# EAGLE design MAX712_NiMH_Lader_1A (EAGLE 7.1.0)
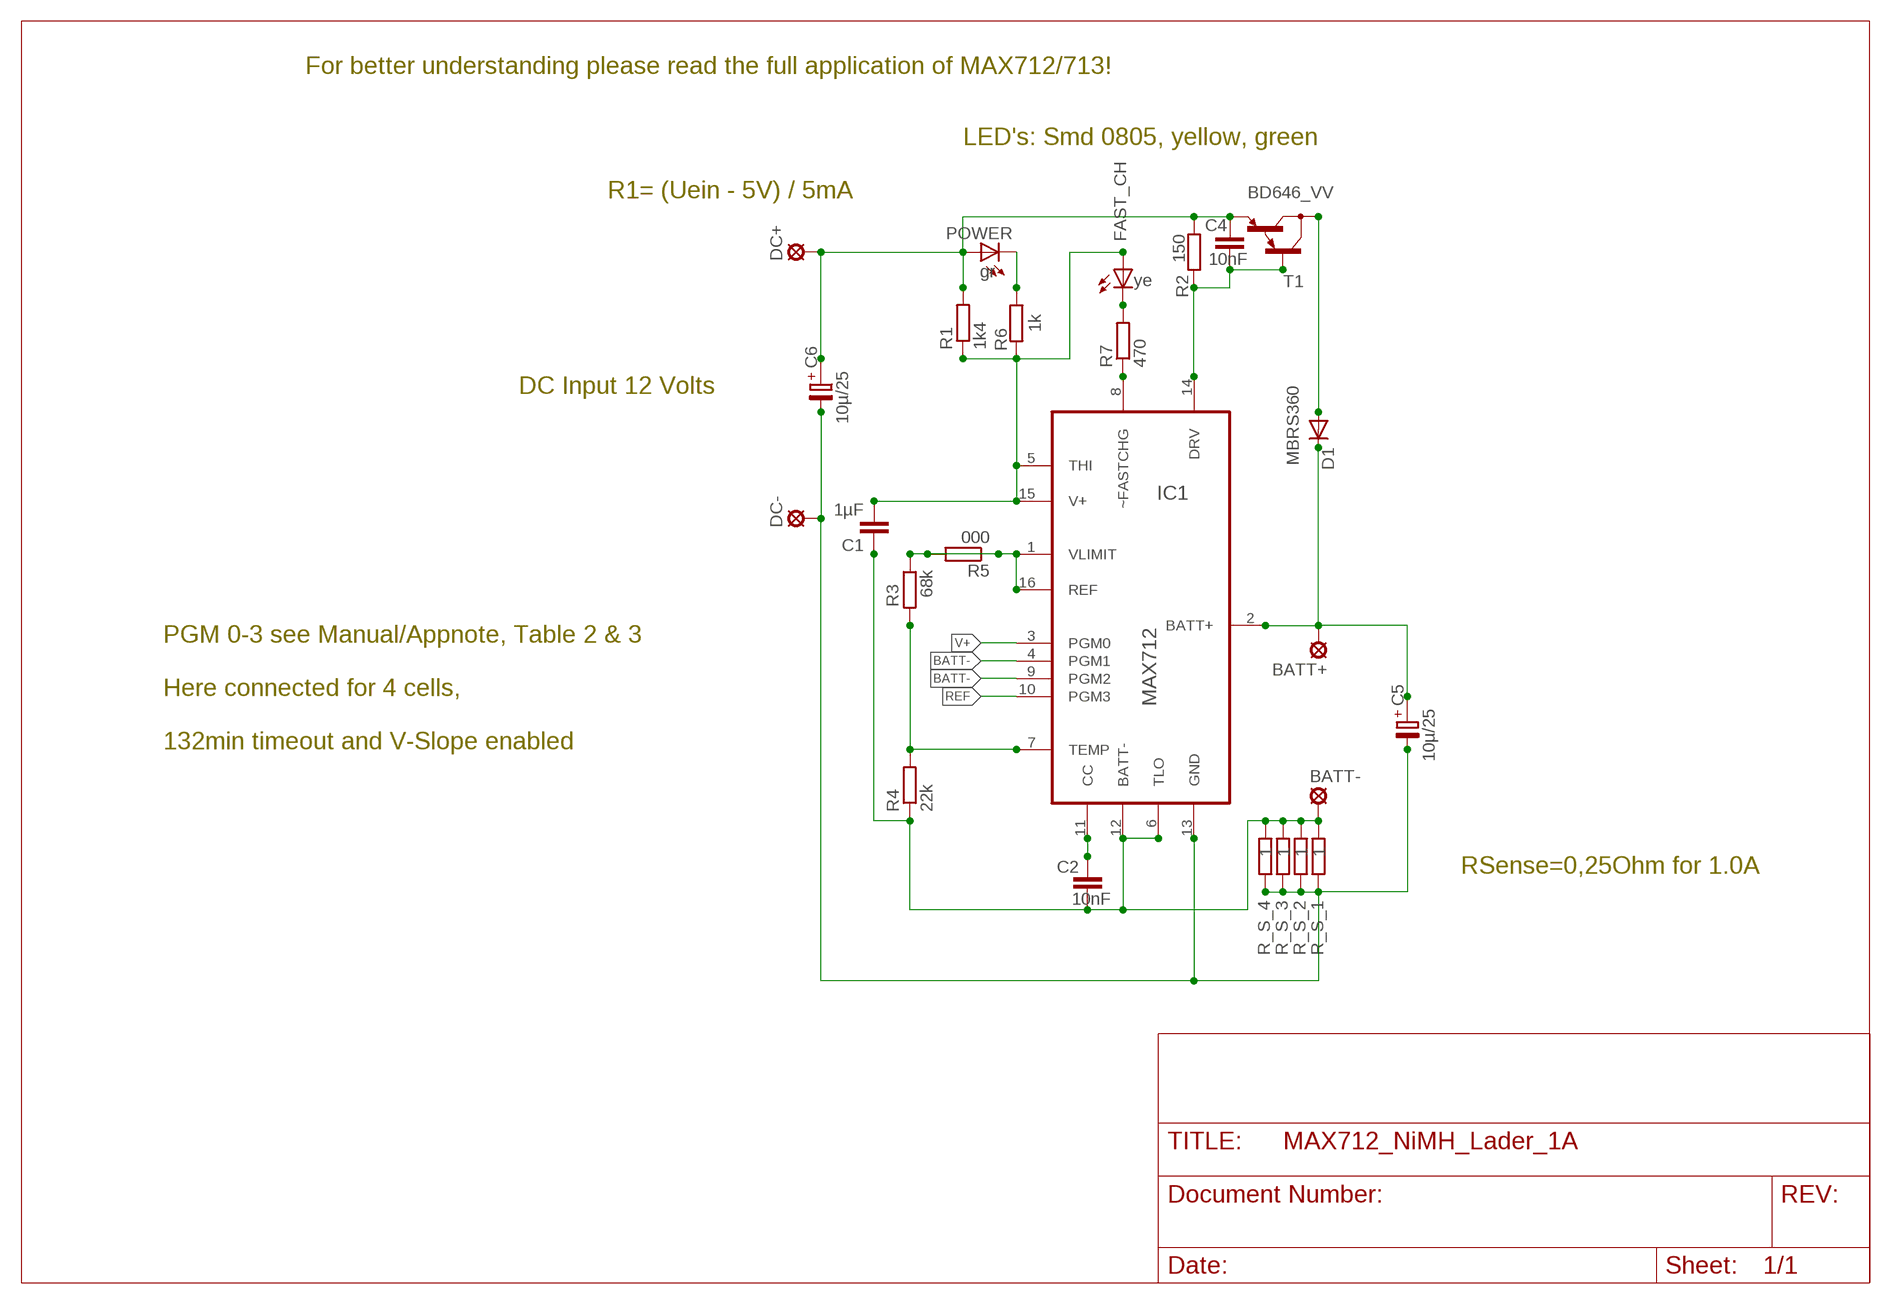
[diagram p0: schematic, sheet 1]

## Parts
BATT+  LSP13  [LSP13]
BATT-  LSP13  [LSP13]
C1  1µF  C-EUC1206  [C1206]
C2  10nF  C-EUC1206  [C1206]
C4  10nF  C-EUC1206  [C1206]
C5  10µ/25  C-PAN-PR-SMD-SV-B  [SV-B]
C6  10µ/25  C-PAN-PR-SMD-SV-B  [SV-B]
D1  MBRS360  MBRS360_SMDSMC  [SMC]
DC+  LSP13  [LSP13]
DC-  LSP13  [LSP13]
FAST_CH  ye  LEDCHIPLED_0805  [CHIPLED_0805]
IC1  MAX712  MAX712_MODDIL16  [DIP254P762X457-16]
POWER  gr  LEDCHIPLED_0805  [CHIPLED_0805]
R1  1k4  R-EU_R1206  [R1206]
R2  150  R-EU_R1206  [R1206]
R3  68k  R-EU_R1206  [R1206]
R4  22k  R-EU_R1206  [R1206]
R5  000  R-EU_R1206  [R1206]
R6  1k  R-EU_R1206  [R1206]
R7  470  R-EU_R1206  [R1206]
R_S_1  1  R-EU_R1206  [R1206]
R_S_2  1  R-EU_R1206  [R1206]
R_S_3  1  R-EU_R1206  [R1206]
R_S_4  1  R-EU_R1206  [R1206]
T1  BD646_VV  [TO220V]

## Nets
BATT+: BATT+.MP C5.+ D1.C IC1.2(BATT+)
BATT-: BATT-.MP C1.1 C2.1 IC1.4(PGM1) IC1.6(TLO) IC1.9(PGM2) IC1.12(BATT-) R4.1 R_S_1.1 R_S_2.1 R_S_3.1 R_S_4.1
CC: C2.2 IC1.11(CC)
DRV: C4.2 IC1.14(DRV) R2.2 T1.1(B)
GND: C5.- C6.- DC-.MP IC1.13(GND) R_S_1.2 R_S_2.2 R_S_3.2 R_S_4.2
N$4: IC1.8(~FASTCHG) R7.1
N$8: POWER.C R6.1
N$9: FAST_CH.C R7.2
N$13: D1.A T1.2(C)
REF: IC1.1(VLIMIT) IC1.10(PGM3) IC1.16(REF) R3.1 R5.1 R5.2
TEMP: IC1.7(TEMP) R3.2 R4.2
V+: C1.2 FAST_CH.A IC1.3(PGM0) IC1.5(THI) IC1.15(V+) R1.1 R6.2
VCC: C4.1 C6.+ DC+.MP POWER.A R1.2 R2.1 T1.3(E)

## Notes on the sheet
- For better understanding please read the full application of MAX712/713!
- LED's: Smd 0805, yellow, green
- R1= (Uein - 5V) / 5mA
- DC Input 12 Volts
- PGM 0-3 see Manual/Appnote, Table 2 & 3
- Here connected for 4 cells,
- 132min timeout and V-Slope enabled
- RSense=0,25Ohm for 1.0A

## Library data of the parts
BATT+ BATT- DC+ DC- = solpad:LSP13: SOLDER PAD
C1 C2 C4 = rcl-kpl:C-EU: CAPACITOR, European symbol
C5 C6 = rcl-kpl:C-PAN-PR: POLARIZED ELECTROLYTIC/TANTALUM
D1 = diode:MBRS360_SMD: SCHOTTKY BARRIER
FAST_CH POWER = led:LED: LED
IC1 = Maxim_By_element14_Batch_1:MAX712_MOD
R1-R7 R_S_1-R_S_4 = rcl-kpl:R-EU_: RESISTOR, European symbol
T1 = transistor-pnp:BD646_V: BD646 - PNP-Darl Uces 60 V Ic 8 A Ptot 62,5 W fT 7 MHz B >750 To220

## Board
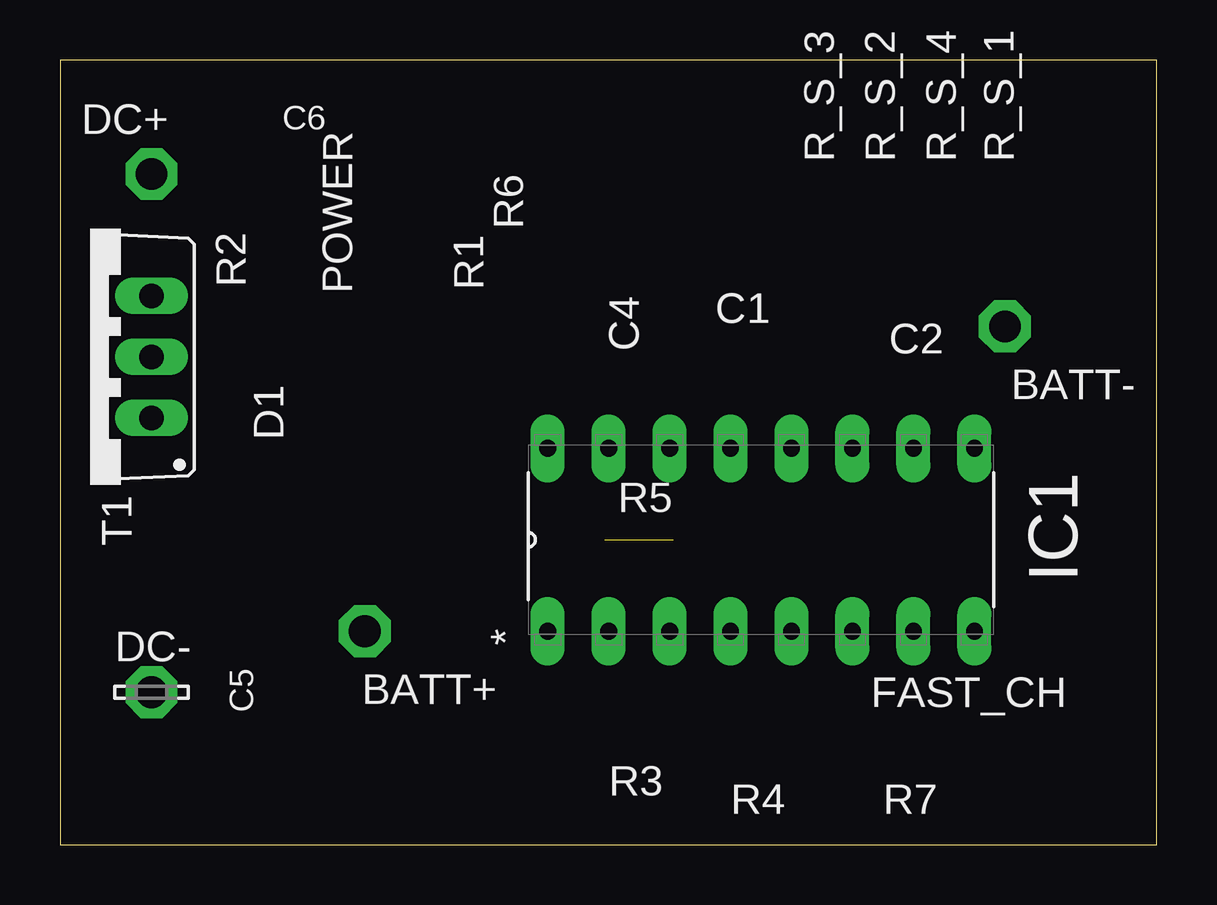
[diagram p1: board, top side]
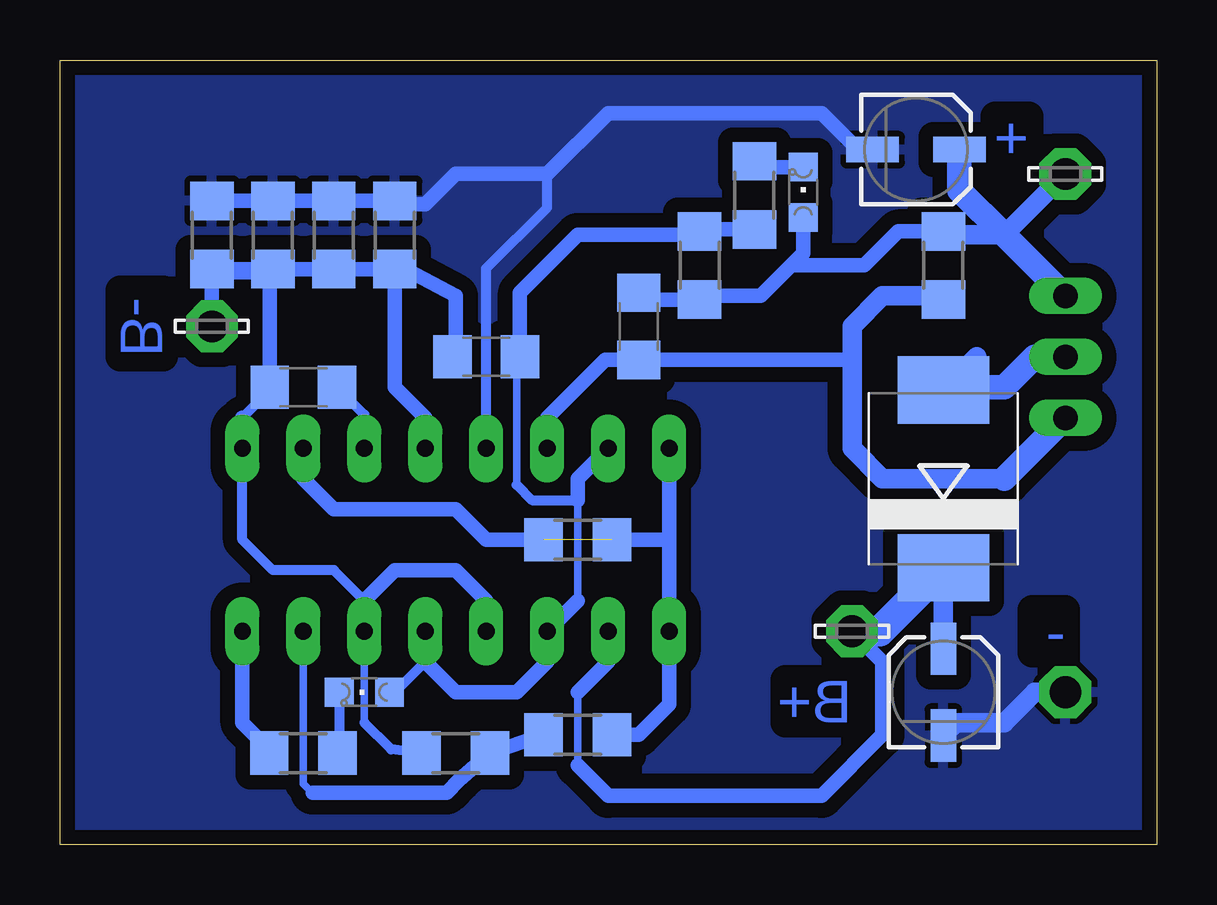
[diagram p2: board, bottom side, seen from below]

Size 45.7 x 32.69 mm. Coordinates in mm from the lower left corner, seen from the top.
Outline: 0,0 45.7,0 45.7,32.69 0,32.69 0,0
Copper layers (1*16): Top 0.035mm / dielectric 1.5mm / Bottom 0.035mm
Design rules "default *": minimum track width 10mil, minimum drill 24mil, track to track 8mil, track to pad 8mil, pad to pad 8mil, via to via 8mil, smd to smd 8mil, copper to edge 10mil, drill to drill 8mil, minimum pad ring 10mil, minimum via ring 8mil, stop-mask expansion 4mil, vias tented up to drill 0mil, thermal gap 10mil
bRestrict: area 25.4,16.5 to 30.5,19.1; area 24.1,12.7 to 29.2,16.5

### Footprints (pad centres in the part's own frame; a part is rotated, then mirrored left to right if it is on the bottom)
LSP13 = drill 1.321 pad 2.159 octagon: MP 0,0
C1206 = smd 1.6 x 1.8: 1 -1.4,0; 2 1.4,0
SV-B = smd 2.184 x 1.067: + -1.81,0; - 1.81,0
SMC = smd 2.8 x 3.8: A 3.7,0; C -3.7,0
CHIPLED_0805 = smd 1.2 x 1.2: A 0,-1.05; C 0,1.05
DIP254P762X457-16 = drill 0.7 pad 1.422 long: 1 -7.62,17.78; 2 -7.62,15.24; 3 -7.62,12.7; 4 -7.62,10.16; 5 -7.62,7.62; 6 -7.62,5.08; 7 -7.62,2.54; 8 -7.62,0; 9 0,0; 10 0,2.54; 11 0,5.08; 12 0,7.62; 13 0,10.16; 14 0,12.7; 15 0,15.24; 16 0,17.78
R1206 = smd 1.6 x 1.803: 1 -1.422,0; 2 1.422,0
TO220V = drill 1.016 long: 1 -2.54,-2.54; 2 0,-2.54; 3 2.54,-2.54

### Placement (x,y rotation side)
BATT+  12.7,8.89 0 bottom
BATT-  39.37,21.59 0 bottom
C1  27.94,20.32 0 bottom
C2  35.56,19.05 0 bottom
C4  21.59,21.59 270 bottom
C5  8.89,6.35 270 bottom
C6  10.03,28.96 180 bottom
D1  8.89,15.24 90 bottom
DC+  3.81,27.94 0 bottom
DC-  3.81,6.35 0 top
FAST_CH  33.02,6.35 90 bottom
IC1  38.1,16.51 90 top
POWER  14.73,27.18 0 bottom
R1  19.05,24.13 270 bottom
R2  8.89,24.13 270 bottom
R3  24.13,4.57 180 bottom
R4  29.21,3.81 0 bottom
R5  24.13,12.7 0 bottom
R6  16.76,27.05 270 bottom
R7  35.56,3.81 0 bottom
R_S_1  39.37,25.4 90 bottom
R_S_2  34.29,25.4 90 bottom
R_S_3  31.75,25.4 90 bottom
R_S_4  36.83,25.4 90 bottom
T1  1.27,20.32 90 top

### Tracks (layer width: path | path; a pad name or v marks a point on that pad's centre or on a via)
BATT+
  Bottom 0.305: 24.13,3.3 24.13,6.35
  Bottom 0.61: 24.13,3.3 22.86,2.03 13.97,2.03 11.43,4.57 11.43,7.62 BATT+.MP | 24.13,6.35 22.86,7.62 IC1.2
  Bottom 0.813: C5.+ D1.C
  Bottom 1.27: BATT+.MP 11.54,8.89 D1.C
BATT-
  Bottom 0.305: 33.02,5.08 IC1.6
  Bottom 0.406: R4.1 31.9,3.96 33.02,5.08 | 33.02,10.16 34.29,11.43 36.83,11.43 38.1,12.7 IC1.9 | C2.1 36.96,18.92 38.1,17.78
  Bottom 0.61: C1.1 29.21,20.45 29.21,22.86 31.6,24.13 R_S_3.1 | IC1.9 38.1,17.78 | IC1.4 27.94,10.16 29.21,11.43 31.75,11.43 33.02,10.16 IC1.6 | R_S_3.1 R_S_2.1 R_S_4.1 | R_S_4.1 R_S_1.1 | R_S_1.1 39.52,23.98 | C2.1 36.96,23.85 | 36.96,23.85 R_S_4.1 | IC1.12 30.48,17.78 31.75,19.05 R_S_3.1 | 36.96,23.85 39.09,23.85 39.37,24.13 | BATT-.MP R_S_1.1
CC
  Bottom 0.406: IC1.11 33.02,17.91 C2.2
DRV
  Bottom 0.61: IC1.14 25.4,17.78 22.99,20.19 C4.2 12.83,20.19 12.7,20.32
  Bottom 0.813: 6.35,15.24 11.43,15.24 12.7,16.51 12.7,20.32 12.7,21.59 11.43,22.86 9.04,22.86 R2.2
  Bottom 1.016: 6.35,15.24 T1.1
GND
  Bottom 0.406: IC1.13 27.94,24 25.4,26.54 25.4,27.94
  Bottom 0.61: R_S_1.2 R_S_4.2 R_S_2.2 R_S_3.2 31.6,26.67 30.48,26.67 29.21,27.94 25.4,27.94 22.86,30.48 13.97,30.48 12.45,28.96 C6.-
  Bottom 0.813: DC-.MP 5.08,6.35 6.35,5.08 8.35,5.08 C5.-
  pour Bottom (isolate 0.61): 0,0 0,33.02 45.72,33.02 45.72,0
N$4
  Bottom 0.61: R7.1 36.98,3.96 38.1,5.08 IC1.8
N$8
  Bottom 0.61: POWER.C 16.52,28.23 R6.1
N$9
  Bottom 0.406: FAST_CH.C 34.07,3.88 R7.2
N$13
  Bottom 0.813: 7.51,20.32 D1.A
  Bottom 1.016: T1.2 5.08,20.32 6.35,19.05 8.78,19.05 D1.A
REF  (1 unrouted)
  Bottom 0.61: R3.1 21.59,4.57 20.32,5.84 IC1.1 20.32,12.7 | 20.32,12.7 IC1.16 | R5.2 20.32,12.7 | R5.1 27.94,12.7 29.21,13.97 34.29,13.97 35.56,15.24 IC1.10
TEMP
  Bottom 0.305: 35.18,2.16 35.56,2.54 IC1.7
  Bottom 0.61: R3.2 R4.2 29.06,2.69 29.59,2.16 35.18,2.16
V+
  Bottom 0.305: 24.13,10.16 24.13,14.35 | 26.67,20.19 26.67,14.99
  Bottom 0.406: FAST_CH.A 31.75,6.35 30.48,7.62 | 26.67,14.99 26.04,14.35 24.13,14.35
  Bottom 0.61: IC1.5 30.48,7.62 29.21,6.35 26.67,6.35 25.4,7.62 IC1.3 24.13,10.16 | 24.13,14.35 24.13,15.24 IC1.15 | 26.67,20.32 26.67,20.19 C1.2 26.54,22.99 24.13,25.4 19.05,25.4 R1.1 18.97,25.63 R6.2
VCC
  Bottom 0.61: R2.1 10.77,25.55 12.19,24.13 15.24,24.13 | 15.24,24.13 16.51,22.86 18.9,22.86 R1.2 21.31,22.71 C4.1 | POWER.A 14.73,24.64 15.24,24.13
  Bottom 0.813: R2.1 8.74,25.4 6.35,25.4 DC+.MP
  Bottom 1.016: T1.3 6.35,25.4 8.22,27.27 C6.+

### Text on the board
Bottom: + | B- | - | B+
